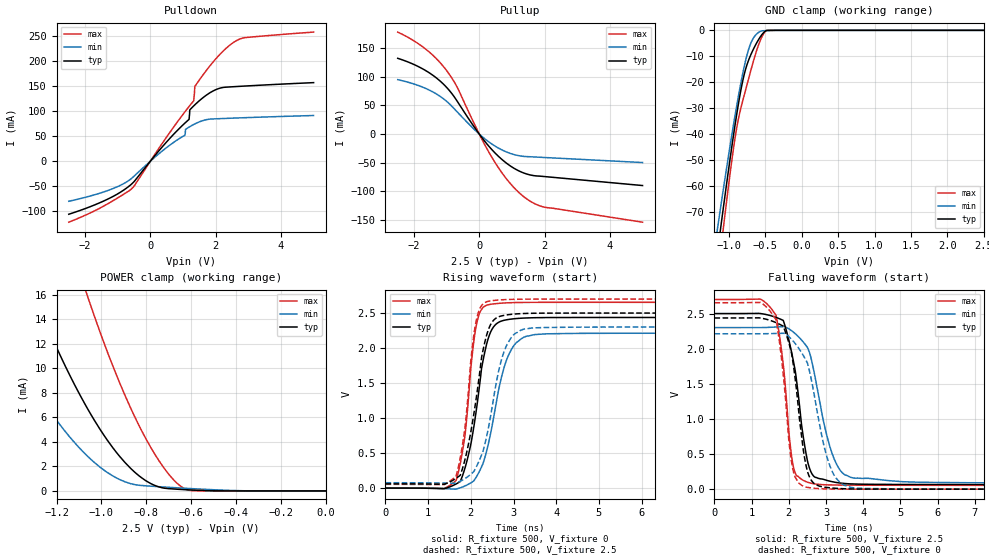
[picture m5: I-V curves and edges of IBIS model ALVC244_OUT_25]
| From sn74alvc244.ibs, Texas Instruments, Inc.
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[Model]   ALVC244_OUT_25
Model_type  3-state
Enable   Active-Low
Vref =   0
Rref =   500
Cref =   30p
Vmeas =   1.25
| variable   typ   min   max
C_comp   6.27pF   5.57pF   7.18pF
| C_pullup   8.59pF   6.26pF   10.00pF
| C_pulldown   11.89pF   0.71pF   28.20pF
| C_tri-state   6.27pF   5.57pF   7.18pF
[Temperature Range]   40   100   -40
| Ambient temperature   25   85   -40
[Voltage range]   2.5   2.3   2.7
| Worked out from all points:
|   slope of the pulldown table from 0 to 0.375 V, typ, clamps not added: 12.8 ohm
|   slope of the pullup table from 0 to 0.375 V, typ, clamps not added: 14.2 ohm
|   GND clamp passes 1 mA (typ) near -0.53 V on its own axis
|   POWER clamp passes 1 mA (typ) near -0.82 V on its own axis
|   rising waveform, R_fixture 500, V_fixture 0: 20-80 % time 381ps typ, 472ps min, 269ps max; typ from 0 V to 2.44 V
|   falling waveform, R_fixture 500, V_fixture 2.5: 20-80 % time 401ps typ, 554ps min, 294ps max; typ from 2.5 V to 0.061 V
|   rising waveform, R_fixture 500, V_fixture 2.5: 20-80 % time 384ps typ, 448ps min, 272ps max; typ from 0.061 V to 2.5 V
|   falling waveform, R_fixture 500, V_fixture 0: 20-80 % time 342ps typ, 521ps min, 295ps max; typ from 2.44 V to 0 V
[GND Clamp]
| ALVC244_OUT_25
|   Voltage   I(typ)   I(min)   I(max)
-2.5V     -398.6mA   -355.1mA   -442.4mA
-1.155V   -84.62mA   -75.62mA   -94.35mA
-1.125V   -78.21mA   -69.94mA   -87.17mA
-1.095V   -71.87mA   -64.33mA   -80.07mA
-1.07V    -66.64mA   -59.7mA    -74.23mA
-915mV    -36.06mA   -32.44mA   -41.08mA
-870mV    -28.2mA    -25.22mA   -33.97mA
-810mV    -19.28mA   -16.44mA   -26.95mA
-705mV    -9.7mA     -5.291mA   -15.94mA
-575mV    -2.729mA   -487.5uA   -4.215mA
-475mV    -33.84uA   -89.41uA   -29.91uA
2.5V      99.58pA    107.2nA    13.28pA
[POWER Clamp]
| ALVC244_OUT_25
|   Voltage   I(typ)   I(min)   I(max)
-2.5V     91.01mA    61.46mA    135.5mA
-1.535V   27.58mA    16.2mA     47.67mA
-1.515V   26.5mA     15.47mA    46.12mA
-1.295V   15.71mA    8.296mA    30.16mA
-1.165V   10.33mA    4.931mA    21.81mA
-1.06V    6.645mA    2.798mA    15.77mA
-950mV    3.54mA     1.231mA    10.22mA
-845mV    1.423mA    493.2uA    5.796mA
-745mV    332.8uA    345.7uA    2.502mA
-655mV    131.2uA    246.7uA    499.2uA
-595mV    72.53uA    185.3uA    21.89uA
-31.15fV  99.58pA    519.4pA    14.82pA
[Pulldown]
| ALVC244_OUT_25
|   Voltage   I(typ)   I(min)   I(max)
-2.5V     -105.7mA   -79.86mA   -121.5mA
-540mV    -43.43mA   -32.24mA   -52.78mA
1.06V     75.89mA    51.69mA    98.32mA
1.185V    83.13mA    67.78mA    108.8mA
1.21V     102.2mA    68.76mA    110.8mA
1.305V    108.5mA    72.27mA    118.5mA
1.33V     110.1mA    73.13mA    120.2mA
1.365V    112.3mA    74.29mA    149mA
1.94V     140.3mA    84.09mA    198.8mA
2.445V    147.8mA    85.43mA    231.5mA
2.885V    149.5mA    86.51mA    245.8mA
5V        156.3mA    90.86mA    256.9mA
[Pullup]
| ALVC244_OUT_25
|   Voltage   I(typ)   I(min)   I(max)
-2.5V     132.3mA    95.07mA    178mA
-1.665V   111.6mA    80.27mA    149.3mA
-1.325V   98.46mA    70.4mA     132.2mA
-1.025V   82.92mA    58.34mA    112.6mA
-680mV    57.59mA    38.9mA     82mA
30mV      -2.342mA   -1.535mA   -3.449mA
440mV     -30.41mA   -19.35mA   -45.74mA
910mV     -53.92mA   -32.83mA   -83.53mA
1.38V     -68.18mA   -38.91mA   -110mA
1.69V     -72.54mA   -39.83mA   -121.2mA
2.005V    -74.04mA   -40.76mA   -127.5mA
5V        -89.66mA   -49.55mA   -153.6mA
[Ramp]
| ALVC244_OUT_25
| variable   typ   min   max
dV/dt_r   1.47/4.02E-10   1.34/4.95E-10   1.60/2.86E-10
dV/dt_f   1.47/4.32E-10   1.34/5.72E-10   1.59/3.13E-10
R_load = 500
[Rising Waveform]
| ALVC244_OUT_25
R_fixture =   500
C_fixture =   0
L_fixture =   0
V_fixture =   0
V_fixture_min = 0
V_fixture_max = 0
|   Time   V(typ)   V(min)   V(max)
0s        60.07pV    3.608nV    48.12pV
1.655ns   58.99mV    -12.84mV   109.8mV
1.865ns   291.5mV    30.91mV    762.2mV
2.02ns    694.1mV    82.63mV    1.833V
2.15ns    1.209V     181.2mV    2.385V
2.375ns   2.068V     542.6mV    2.613V
2.68ns    2.377V     1.486V     2.64V
3.04ns    2.421V     2.061V     2.65V
3.79ns    2.436V     2.204V     2.654V
50ns      2.437V     2.212V     2.654V
[Falling Waveform]
| ALVC244_OUT_25
R_fixture =   500
C_fixture =   0
L_fixture =   0
V_fixture =   2.5
V_fixture_min = 2.3
V_fixture_max = 2.7
|   Time   V(typ)   V(min)   V(max)
0s        2.5V       2.3V       2.7V
1.41ns    2.484V     2.302V     2.639V
1.66ns    2.444V     2.308V     2.466V
1.85ns    2.402V     2.315V     1.772V
2.145ns   1.76V      2.226V     271.5mV
2.5ns     403mV      2.018V     99.49mV
2.79ns    154.3mV    1.361V     68.88mV
3.435ns   83.87mV    234.4mV    58.06mV
5.07ns    67.02mV    106mV      55.65mV
50ns      60.54mV    76.66mV    53.33mV
[Rising Waveform]
| ALVC244_OUT_25
R_fixture =   500
C_fixture =   0
L_fixture =   0
V_fixture =   2.5
V_fixture_min = 2.3
V_fixture_max = 2.7
|   Time   V(typ)   V(min)   V(max)
0s        60.54mV    76.63mV    53.33mV
1.655ns   139.9mV    73.24mV    173.7mV
1.865ns   414.2mV    136.4mV    877.3mV
2.01ns    839.6mV    203.4mV    1.883V
2.14ns    1.344V     317.5mV    2.43V
2.365ns   2.173V     724.3mV    2.661V
2.63ns    2.441V     1.61V      2.686V
2.99ns    2.484V     2.182V     2.696V
3.695ns   2.499V     2.293V     2.7V
50ns      2.5V       2.3V       2.7V
[Falling Waveform]
| ALVC244_OUT_25
R_fixture =   500
C_fixture =   0
L_fixture =   0
V_fixture =   0
V_fixture_min = 0
V_fixture_max = 0
|   Time   V(typ)   V(min)   V(max)
0s        2.437V     2.212V     2.654V
1.42ns    2.415V     2.213V     2.58V
1.66ns    2.37V      2.216V     2.401V
1.85ns    2.32V      2.219V     1.63V
2.135ns   1.718V     2.096V     224.5mV
2.425ns   439.3mV    1.87V      36.24mV
2.68ns    80.2mV     1.352V     13.05mV
3.175ns   15.98mV    241.9mV    1.872mV
3.885ns   1.595mV    12mV       103.8uV
50ns      484.3nV    2.657uV    272nV
